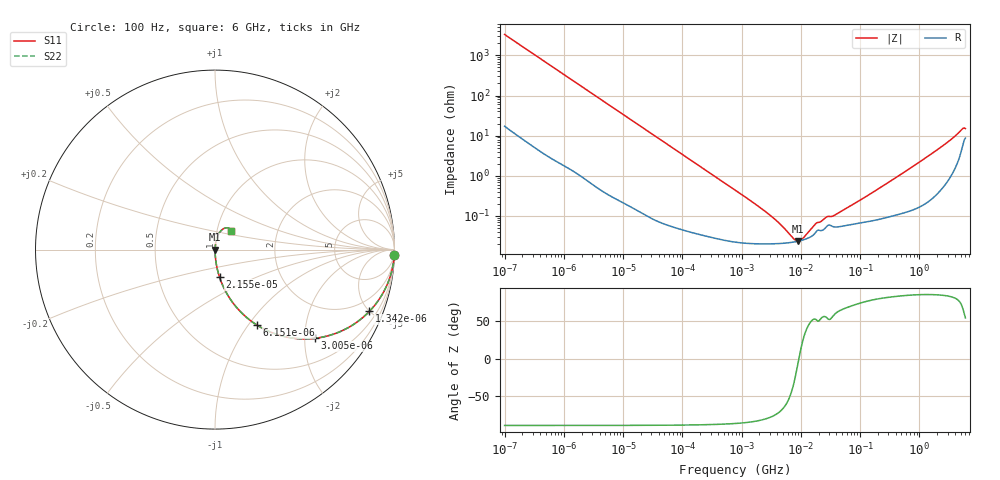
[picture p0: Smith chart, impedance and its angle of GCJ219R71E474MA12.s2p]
!Murata Part Number: GCJ219R71E474MA12
!These Parameters are Measured in Series Mode Connection
!Data Generated on Mar 13, 2026
!  o--ll--o
!Port1  Port2
!  o------o
!Operation Temp=25[degC], DC Bias Voltage=0[V]
!Freq. Start=100[Hz] Stop=6[GHz] 401[Steps]
# Hz S RI R 50
!Freq.(Hz) S11(Real) S11(Imag) S21(Real) S21(Imag) S12(Real) S12(Imag) S22(Real) S22(Imag)
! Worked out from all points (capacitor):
!   401 points, 100 Hz to 6 GHz, reference 50 ohm
!   read as one part in series: C = 478 nF near 109 Hz
!   lowest |Z| = 23.5 mohm at 9.09 MHz (marker M1)
!   series resonance near 9.286 MHz, so ESL is about 610 pH
!   S11 on the Smith chart (normalised r, x): 100 Hz: 1, -67; 1.342 kHz: 1.03, -5.00; 3.005 kHz: 1.01, -2.24; 6.151 kHz: 1.01, -1.10; 21.55 kHz: 1.00, -0.31; 6 GHz: 1.17, +0.24
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100  0.9989 -0.03  0.00106 0.03  0.00106 0.03  0.9989 -0.03
419  0.9839 -0.1233  0.0161 0.1233  0.0161 0.1233  0.9839 -0.1233
820  0.9423 -0.2306  0.0577 0.2306  0.0577 0.2306  0.9423 -0.2306
1342  0.8605 -0.3437  0.1395 0.3437  0.1395 0.3437  0.8605 -0.3437
2008  0.7355 -0.4383  0.2645 0.4383  0.2645 0.4383  0.7355 -0.4383
3005  0.5558 -0.4941  0.4442 0.4941  0.4442 0.4941  0.5558 -0.4941
6151  0.2322 -0.4194  0.7678 0.4194  0.7678 0.4194  0.2322 -0.4194
10527  0.0948 -0.2898  0.9052 0.2898  0.9052 0.2898  0.0948 -0.2898
21550  0.0251 -0.153  0.9749 0.153  0.9749 0.153  0.0251 -0.153
40335  0.00772 -0.0834  0.9923 0.0834  0.9923 0.0834  0.00772 -0.0834
774597  0.000241 -0.00442  0.9998 0.00442  0.9998 0.00442  0.000241 -0.00442
2967816  0.000201 -0.00104  0.9998 0.00104  0.9998 0.00104  0.000201 -0.00104
7599586  0.000223 -0.000149  0.9998 0.000149  0.9998 0.000149  0.000223 -0.000149
9090158  0.000235 -1.55e-05  0.9998 1.55e-05  0.9998 1.55e-05  0.000235 -1.55e-05
1.087309e7  0.000251 0.000116  0.9997 -0.000116  0.9997 -0.000116  0.000251 0.000116
1.555665e7  0.000317 0.000396  0.9997 -0.000396  0.9997 -0.000396  0.000317 0.000396
2.662322e7  0.00052 0.000759  0.9995 -0.000759  0.9995 -0.000759  0.00052 0.000759
3.80911e7  0.000527 0.000922  0.9995 -0.000922  0.9995 -0.000922  0.000527 0.000922
3.124326e8  0.000994 0.00699  0.999 -0.00699  0.999 -0.00699  0.000994 0.00699
3.065283e9  0.0123 0.0685  0.9877 -0.0685  0.9877 -0.0685  0.0123 0.0685
5.245841e9  0.0613 0.1216  0.9387 -0.1216  0.9387 -0.1216  0.0613 0.1216
6e9  0.0914 0.1022  0.9086 -0.1022  0.9086 -0.1022  0.0914 0.1022
